| TEXAS INSTRUMENTS INCORPORATED
| Standard Linear and Logic Group
| IBIS Model of SN74ALVCH16501
| 18-BIT UNIVERSAL BUS TRANSCEIVER WITH 3-STATE OUTPUTS
| This file contains package information for the following:
|  TSSOP 56-pin (DGG) package as [Component] ALVCH16501_DGG
|  SSOP 56-pin (DL) package as [Component] ALVCH16501_DL
|  VFBGA 56-pin (GQL) package as [Component] ALVCH16501_GQL
| This device can be powered at the following Vccs:
|  1.8 volt Vcc
|  2.5 volt Vcc
|  3.3 volt Vcc
| This file provides unique models under the [Model Selector] for each Vcc.
| For operation at a specific Vcc, select the appropriate model after each
| [Model Selector] keyword.
[IBIS Ver]   3.2
[Comment char]  |_char
[File Name]   sn74alvch16501.ibs
[File Rev]   2.2 | b_die
[Date]   April 19, 2003
[Source]   Data created from TI-SPICE simulations at TI-SLL.
[Notes]   The following is an IBIS list for the ALVCH16501.
   Please contact sllibis@ti.com with questions and
   comments concerning SLL IBIS models.
   - FILE REV HISTORY
   - 2.2 VIH and VIL numbers changed on 04/19/04
   - Non-monotonic data in GND clamp due to bus-hold
   - C_comp values are taken at a different test condition
   than the data sheet.
   - Power clamp data has been deleted in the control pins
   as there is no power-clamp diode in control pins.
[Disclaimer] Property of Texas Instruments Incorporated.  Unauthorized
   reproduction and/or distribution is strictly prohibited.
   This product is protected under copyright law.
   Created  2002, (C) Copyright  2002, Texas Instruments
   Incorporated, All Rights Reserved
   UNLESS THERE IS A SIGNED, WRITTEN AGREEMENT TO THE
   CONTRARY, TEXAS INSTRUMENTS (TI) IS PROVIDING THE IBIS
   MODELS  AND WITHOUT ANY WARRANTY, EXPRESSED OR
   IMPLIED.  TI assumes no liability for:
   1) the accuracy of the IBIS models provided to your
   company;
   2) the proper functioning of these IBIS Models in your
   design or for any resulting applications; or
   3) infringement of patents, copyrights or intellectual
   property rights resulting from your use of these IBIS
   models.
   TI provides IBIS Models as a service to our customers.
   You and your company shall not distribute, sell or give
   these models to anyone else without prior written
   permission from TI.
   TI reserves the right to make changes to our products or
   to discontinue any semiconductor product or service
   without notice, and advises our customers to obtain the
   latest version of relevant information to verify, before
   placing orders, that the information being relied on is
   current.
   Please be aware that your receipt and use of the IBIS
   information provided shall serve as acceptance of these
   terms and conditions.  If you do not accept these terms,
   you should return or destroy the IBIS models and any
   other accompanying information immediately.
| Component ALVCH16501_DGG 56-pin TSSOP
[Component]   ALVCH16501_DGG
[Manufacturer]   Texas Instruments, Inc.
[Package]
|   typ   min   max
R_pkg   4.500e-02   3.500e-02   6.200e-02
L_pkg   3.324e-09   2.403e-09   5.094e-09
C_pkg   5.640e-13   3.410e-13   9.140e-13
[Pin]   signal_name   model_name   R_pin   L_pin   C_pin
1   OEAB   ALVCH16501_OE   6.200e-02   5.094e-09   8.560e-13
2   LEAB   ALVCH16501_LE   6.100e-02   4.621e-09   9.020e-13
3   A1   ALVCH16501_IO   6.000e-02   4.316e-09   8.020e-13
4   GND   GND   5.900e-02   3.968e-09   6.980e-13
5   A2   ALVCH16501_IO   5.700e-02   3.716e-09   6.490e-13
6   A3   ALVCH16501_IO   4.200e-02   3.517e-09   6.520e-13
7   VCC   POWER   4.100e-02   3.160e-09   5.700e-13
8   A4   ALVCH16501_IO   3.900e-02   2.981e-09   4.820e-13
9   A5   ALVCH16501_IO   3.900e-02   2.809e-09   4.470e-13
10   A6   ALVCH16501_IO   3.800e-02   2.715e-09   4.090e-13
11   GND   GND   4.100e-02   2.675e-09   3.910e-13
12   A7   ALVCH16501_IO   3.900e-02   2.536e-09   3.660e-13
13   A8   ALVCH16501_IO   3.900e-02   2.457e-09   3.480e-13
14   A9   ALVCH16501_IO   3.800e-02   2.411e-09   3.530e-13
15   A10   ALVCH16501_IO   3.900e-02   2.456e-09   3.550e-13
16   A11   ALVCH16501_IO   3.900e-02   2.471e-09   3.490e-13
17   A12   ALVCH16501_IO   4.000e-02   2.580e-09   3.700e-13
18   GND   GND   3.800e-02   2.651e-09   3.890e-13
19   A13   ALVCH16501_IO   3.800e-02   2.739e-09   4.110e-13
20   A14   ALVCH16501_IO   3.900e-02   2.838e-09   4.490e-13
21   A15   ALVCH16501_IO   3.800e-02   2.988e-09   4.840e-13
22   VCC   POWER   3.800e-02   3.105e-09   5.640e-13
23   A16   ALVCH16501_IO   4.000e-02   3.427e-09   6.380e-13
24   A17   ALVCH16501_IO   5.600e-02   3.654e-09   6.410e-13
25   GND   GND   5.700e-02   3.932e-09   7.000e-13
26   A18   ALVCH16501_IO   5.800e-02   4.257e-09   8.060e-13
27   NOEBA   ALVCH16501_OE   5.700e-02   4.580e-09   9.140e-13
28   LEBA   ALVCH16501_LE   5.900e-02   5.038e-09   8.610e-13
29   GND   GND   6.000e-02   5.058e-09   8.580e-13
30   CLKBA   ALVCH16501_CLK   5.600e-02   4.543e-09   9.040e-13
31   B18   ALVCH16501_IO   5.700e-02   4.240e-09   8.030e-13
32   GND   GND   5.700e-02   3.929e-09   7.000e-13
33   B17   ALVCH16501_IO   5.600e-02   3.616e-09   6.370e-13
34   B16   ALVCH16501_IO   3.700e-02   3.368e-09   6.400e-13
35   VCC   POWER   3.600e-02   3.024e-09   5.630e-13
36   B15   ALVCH16501_IO   3.500e-02   2.876e-09   4.740e-13
37   B14   ALVCH16501_IO   3.500e-02   2.745e-09   4.440e-13
38   B13   ALVCH16501_IO   3.700e-02   2.683e-09   4.050e-13
39   GND   GND   3.800e-02   2.603e-09   3.820e-13
40   B12   ALVCH16501_IO   3.800e-02   2.510e-09   3.620e-13
41   B11   ALVCH16501_IO   3.600e-02   2.412e-09   3.410e-13
42   B10   ALVCH16501_IO   3.800e-02   2.416e-09   3.490e-13
43   B9   ALVCH16501_IO   3.700e-02   2.403e-09   3.490e-13
44   B8   ALVCH16501_IO   3.700e-02   2.429e-09   3.410e-13
45   B7   ALVCH16501_IO   3.600e-02   2.482e-09   3.580e-13
46   GND   GND   3.700e-02   2.615e-09   3.810e-13
47   B6   ALVCH16501_IO   3.500e-02   2.669e-09   4.020e-13
48   B5   ALVCH16501_IO   3.600e-02   2.763e-09   4.420e-13
49   B4   ALVCH16501_IO   3.600e-02   2.942e-09   4.780e-13
50   VCC   POWER   3.500e-02   3.053e-09   5.640e-13
51   B3   ALVCH16501_IO   3.600e-02   3.409e-09   6.410e-13
52   B2   ALVCH16501_IO   5.800e-02   3.698e-09   6.410e-13
53   GND   GND   5.900e-02   3.975e-09   6.970e-13
54   B1   ALVCH16501_IO   6.100e-02   4.327e-09   8.020e-13
55   CLKAB   ALVCH16501_CLK   6.100e-02   4.624e-09   9.050e-13
56   GND   GND   6.000e-02   5.063e-09   8.580e-13
| Component ALVCH16501_DL 56-pin SSOP
[Component]   ALVCH16501_DL
[Manufacturer]   Texas Instruments, Inc.
[Package]
|   typ   min   max
R_pkg   5.500e-02   4.800e-02   6.700e-02
L_pkg   6.539e-09   4.802e-09   9.746e-09
C_pkg   1.880e-13   7.600e-14   5.170e-13
[Pin]   signal_name   model_name   R_pin   L_pin   C_pin
1   OEAB   ALVCH16501_OE   6.400e-02   9.646e-09   5.130e-13
2   LEAB   ALVCH16501_LE   5.900e-02   8.723e-09   2.700e-13
3   A1   ALVCH16501_IO   5.900e-02   8.139e-09   2.230e-13
4   GND   GND   5.600e-02   7.554e-09   2.010e-13
5   A2   ALVCH16501_IO   5.400e-02   6.991e-09   1.950e-13
6   A3   ALVCH16501_IO   5.300e-02   6.659e-09   2.020e-13
7   VCC   POWER   5.500e-02   6.321e-09   2.070e-13
8   A4   ALVCH16501_IO   5.500e-02   5.942e-09   1.330e-13
9   A5   ALVCH16501_IO   5.700e-02   5.767e-09   1.320e-13
10   A6   ALVCH16501_IO   5.400e-02   5.459e-09   1.210e-13
11   GND   GND   5.100e-02   5.224e-09   1.400e-13
12   A7   ALVCH16501_IO   4.800e-02   5.088e-09   1.260e-13
13   A8   ALVCH16501_IO   5.000e-02   5.021e-09   9.600e-14
14   A9   ALVCH16501_IO   5.100e-02   4.802e-09   7.600e-14
15   A10   ALVCH16501_IO   5.100e-02   4.803e-09   7.600e-14
16   A11   ALVCH16501_IO   5.000e-02   5.021e-09   9.600e-14
17   A12   ALVCH16501_IO   4.800e-02   5.088e-09   1.260e-13
18   GND   GND   5.100e-02   5.224e-09   1.400e-13
19   A13   ALVCH16501_IO   5.400e-02   5.459e-09   1.210e-13
20   A14   ALVCH16501_IO   5.700e-02   5.768e-09   1.330e-13
21   A15   ALVCH16501_IO   5.500e-02   5.942e-09   1.330e-13
22   VCC   POWER   5.500e-02   6.320e-09   2.060e-13
23   A16   ALVCH16501_IO   5.300e-02   6.659e-09   2.030e-13
24   A17   ALVCH16501_IO   5.400e-02   6.991e-09   1.960e-13
25   GND   GND   5.600e-02   7.554e-09   2.010e-13
26   A18   ALVCH16501_IO   5.900e-02   8.139e-09   2.230e-13
27   NOEBA   ALVCH16501_OE   5.900e-02   8.727e-09   2.700e-13
28   LEBA   ALVCH16501_LE   6.700e-02   9.746e-09   5.170e-13
29   GND   GND   6.300e-02   9.630e-09   5.110e-13
30   CLKBA   ALVCH16501_CLK   6.000e-02   8.751e-09   2.710e-13
31   B18   ALVCH16501_IO   6.000e-02   8.184e-09   2.250e-13
32   GND   GND   5.600e-02   7.543e-09   2.000e-13
33   B17   ALVCH16501_IO   5.400e-02   7.005e-09   1.960e-13
34   B16   ALVCH16501_IO   5.600e-02   6.714e-09   2.040e-13
35   VCC   POWER   5.800e-02   6.384e-09   2.080e-13
36   B15   ALVCH16501_IO   5.700e-02   5.976e-09   1.340e-13
37   B14   ALVCH16501_IO   5.700e-02   5.743e-09   1.300e-13
38   B13   ALVCH16501_IO   5.400e-02   5.468e-09   1.190e-13
39   GND   GND   5.500e-02   5.328e-09   1.420e-13
40   B12   ALVCH16501_IO   5.200e-02   5.189e-09   1.290e-13
41   B11   ALVCH16501_IO   5.200e-02   5.053e-09   9.600e-14
42   B10   ALVCH16501_IO   5.100e-02   4.825e-09   7.600e-14
43   B9   ALVCH16501_IO   5.400e-02   4.896e-09   7.800e-14
44   B8   ALVCH16501_IO   5.200e-02   5.093e-09   9.700e-14
45   B7   ALVCH16501_IO   5.100e-02   5.179e-09   1.280e-13
46   GND   GND   5.400e-02   5.314e-09   1.420e-13
47   B6   ALVCH16501_IO   5.500e-02   5.511e-09   1.210e-13
48   B5   ALVCH16501_IO   5.700e-02   5.771e-09   1.310e-13
49   B4   ALVCH16501_IO   5.600e-02   5.957e-09   1.330e-13
50   VCC   POWER   5.500e-02   6.320e-09   2.060e-13
51   B3   ALVCH16501_IO   5.200e-02   6.621e-09   2.000e-13
52   B2   ALVCH16501_IO   5.300e-02   6.973e-09   1.950e-13
53   GND   GND   5.700e-02   7.571e-09   2.020e-13
54   B1   ALVCH16501_IO   5.700e-02   8.097e-09   2.220e-13
55   CLKAB   ALVCH16501_CLK   5.900e-02   8.723e-09   2.710e-13
56   GND   GND   6.100e-02   9.560e-09   5.090e-13
|   VFBGA PACKAGE (GQL)
[Component]   ALVCH16501_GQL
[manufacturer]   Texas Instruments, Inc.
[Package]
|   typ   min   max
R_pkg   0.065   0.035   0.097
L_pkg   1.952nH   1.000nH   3.191nH
C_pkg   0.283pF   0.162pF   0.434pF
[Pin] signal_name   model_name   R_pin   L_pin   C_pin
A3   OEAB   ALVCH16501_OE   0.036   1.004nH   0.176pF
A2   LEAB   ALVCH16501_LE   0.04   1.191nH   0.186pF
A1   A1   ALVCH16501_IO   0.047   1.411nH   0.209pF
B3   GND   GND   0.097   3.191nH   0.434pF
B2   A2   ALVCH16501_IO   0.074   2.213nH   0.329pF
B1   A3   ALVCH16501_IO   0.06   1.712nH   0.243pF
C3   VCC   POWER   0.085   2.691nH   0.368pF
C2   A4   ALVCH16501_IO   0.074   2.16nH   0.315pF
C1   A5   ALVCH16501_IO   0.06   1.666nH   0.247pF
D2   A6   ALVCH16501_IO   0.074   2.121nH   0.313pF
D3   GND   GND   0.091   2.924nH   0.397pF
D1   A7   ALVCH16501_IO   0.06   1.619nH   0.245pF
E2   A8   ALVCH16501_IO   0.069   2.031nH   0.288pF
E1   A9   ALVCH16501_IO   0.06   1.583nH   0.22pF
F1   A10   ALVCH16501_IO   0.06   1.578nH   0.22pF
F2   A11   ALVCH16501_IO   0.069   2.017nH   0.286pF
G1   A12   ALVCH16501_IO   0.06   1.594nH   0.241pF
G3   GND   GND   0.092   2.917nH   0.397pF
G2   A13   ALVCH16501_IO   0.075   2.114nH   0.315pF
H1   A14   ALVCH16501_IO   0.06   1.632nH   0.247pF
H2   A15   ALVCH16501_IO   0.07   2.074nH   0.307pF
H3   VCC   POWER   0.086   2.664nH   0.365pF
J1   A16   ALVCH16501_IO   0.06   1.689nH   0.249pF
J2   A17   ALVCH16501_IO   0.066   2.152nH   0.332pF
J3   GND   GND   0.087   3.118nH   0.423pF
K1   A18   ALVCH16501_IO   0.038   1.303nH   0.2pF
K2   NOEBA   ALVCH16501_OE   0.035   1.176nH   0.183pF
K3   LEBA   ALVCH16501_LE   0.035   1.007nH   0.162pF
K4   GND   GND   0.035   1nH   0.162pF
K5   CLKBA   ALVCH16501_CLK   0.035   1.154nH   0.18pF
K6   B18   ALVCH16501_IO   0.041   1.352nH   0.204pF
J4   GND   GND   0.088   3.137nH   0.43pF
J5   B17   ALVCH16501_IO   0.074   2.218nH   0.334pF
J6   B16   ALVCH16501_IO   0.06   1.683nH   0.25pF
H4   VCC   POWER   0.085   2.658nH   0.372pF
H5   B15   ALVCH16501_IO   0.075   2.149nH   0.321pF
H6   B14   ALVCH16501_IO   0.06   1.627nH   0.248pF
G5   B13   ALVCH16501_IO   0.075   2.113nH   0.314pF
G4   GND   GND   0.092   2.922nH   0.396pF
G6   B12   ALVCH16501_IO   0.06   1.594nH   0.242pF
F5   B11   ALVCH16501_IO   0.069   2.016nH   0.288pF
F6   B10   ALVCH16501_IO   0.06   1.58nH   0.221pF
E6   B9   ALVCH16501_IO   0.06   1.582nH   0.22pF
E5   B8   ALVCH16501_IO   0.069   2.026nH   0.289pF
D6   B7   ALVCH16501_IO   0.06   1.61nH   0.245pF
D4   GND   GND   0.092   2.933nH   0.396pF
D5   B6   ALVCH16501_IO   0.075   2.126nH   0.311pF
C6   B5   ALVCH16501_IO   0.06   1.641nH   0.245pF
C5   B4   ALVCH16501_IO   0.073   2.168nH   0.319pF
C4   VCC   POWER   0.086   2.675nH   0.362pF
B6   B3   ALVCH16501_IO   0.06   1.688nH   0.243pF
B5   B2   ALVCH16501_IO   0.075   2.281nH   0.333pF
B4   GND   GND   0.095   3.168nH   0.424pF
A6   B1   ALVCH16501_IO   0.045   1.418nH   0.209pF
A5   CLKAB   ALVCH16501_CLK   0.039   1.216nH   0.19pF
A4   GND   GND   0.037   1.029nH   0.179pF
| Model ALVCH16501_CLK
[Model Selector]   ALVCH16501_CLK
ALVCH16501_CLK_18   1.8 volt Vcc
ALVCH16501_CLK_25   2.5 volt Vcc
ALVCH16501_CLK_33   3.3 volt Vcc
| Model ALVCH16501_OE
[Model Selector]   ALVCH16501_OE
ALVCH16501_OE_18   1.8 volt Vcc
ALVCH16501_OE_25   2.5 volt Vcc
ALVCH16501_OE_33   3.3 volt Vcc
| Model ALVCH16501_LE
[Model Selector]   ALVCH16501_LE
ALVCH16501_LE_18   1.8 volt Vcc
ALVCH16501_LE_25   2.5 volt Vcc
ALVCH16501_LE_33   3.3 volt Vcc
| Model ALVCH16501_IO
[Model Selector]   ALVCH16501_IO
ALVCH16501_IO_18   1.8 volt Vcc
ALVCH16501_IO_25   2.5 volt Vcc
ALVCH16501_IO_33   3.3 volt Vcc
| Models and submodels in the file (12): ALVCH16501_CLK_18 (Input), ALVCH16501_CLK_25 (Input), ALVCH16501_CLK_33 (Input), ALVCH16501_OE_18 (Input), ALVCH16501_OE_25 (Input), ALVCH16501_OE_33 (Input), ALVCH16501_LE_18 (Input), ALVCH16501_LE_25 (Input), ALVCH16501_LE_33 (Input), ALVCH16501_IO_18 (I/O), ALVCH16501_IO_25 (I/O), ALVCH16501_IO_33 (I/O)
